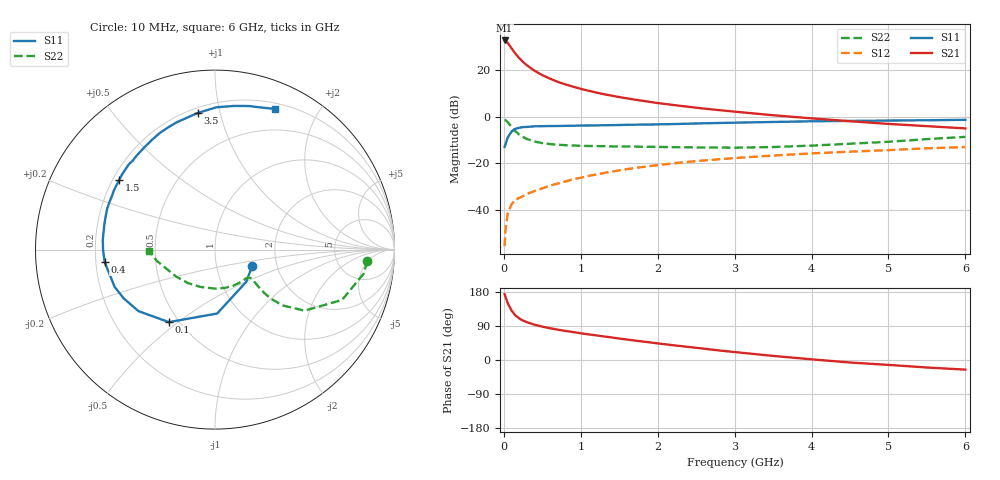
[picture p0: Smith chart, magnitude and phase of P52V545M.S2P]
! SIEMENS Small Signal Semiconductors
! BFP183
! Si NPN RF Bipolar Junction Transistor in SOT143
! VCE = 2.5 V  IC = 45 mA
! Common Emitter S-Parameters:  March  1996
# GHz  S  MA  R  50
!  f  S11  S21  S12  S22
! GHz  MAG  ANG  MAG  ANG  MAG  ANG  MAG  ANG
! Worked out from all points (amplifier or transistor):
!   36 points, 10 MHz to 6 GHz, reference 50 ohm
!   highest |S21| = 32.5 dB at 10 MHz (marker M1)
!   |S21| within 3 dB of that: start of sweep to 92.57 MHz
!   unconditionally stable (mu >= 1): start of sweep to 18.27 MHz; 325 MHz to end of sweep
!   at 250 MHz: K = 0.88, MSG = 28.7 dB, |S12| = -34.0 dB
!   at 1.4 GHz: K = 1.40, MAG = 12.5 dB, |S12| = -23.5 dB
!   at 6 GHz: K = 1.09, MAG = 2.2 dB, |S12| = -13.0 dB
!   S11 on the Smith chart (normalised r, x): 10 MHz: 1.49, -0.29; 100 MHz: 0.44, -0.46; 400 MHz: 0.24, -0.05; 1.5 GHz: 0.23, +0.31; 3.5 GHz: 0.23, +0.85; 6 GHz: 0.26, +1.48
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0.01  0.2264 -24.0  42.32 173.6  0.0017 76.9  0.8506 -4.3
0.02  0.2502 -45.8  41.79 167.6  0.0036 69.7  0.8397 -9.1
0.05  0.3565 -88.1  37.76 150.3  0.0085 68.6  0.7616 -21.6
0.1  0.4789 -122.5  28.78 130.3  0.0133 53.8  0.6038 -34.3
0.15  0.5472 -141.2  22.26 117.9  0.0168 50.5  0.4877 -39.6
0.2  0.5771 -152.0  17.81 109.7  0.0182 50.2  0.413 -41.3
0.25  0.5968 -159.7  14.7 103.9  0.02 50.4  0.3659 -41.4
0.3  0.6009 -165.4  12.45 99.8  0.0222 51.4  0.3318 -40.8
0.4  0.619 -173.6  9.535 93.0  0.0256 54.1  0.2926 -39.6
0.5  0.6238 179.9  7.675 88.1  0.0292 55.4  0.2713 -38.9
0.6  0.6276 174.9  6.473 83.8  0.0334 58.1  0.2585 -38.6
0.7  0.6292 170.1  5.524 80.1  0.037 59.5  0.2502 -38.9
0.9  0.6369 162.9  4.35 73.8  0.0458 60.6  0.2408 -40.7
1.1  0.6451 155.7  3.565 67.6  0.054 60.6  0.235 -43.6
1.5  0.6594 144.2  2.61 56.6  0.0708 58.9  0.2298 -51.2
1.8  0.6757 135.1  2.178 48.8  0.0836 56.9  0.226 -58.5
2.2  0.6914 125.1  1.768 39.0  0.0998 53.2  0.2216 -69.0
2.8  0.7292 111.0  1.373 25.1  0.1225 47.3  0.2178 -87.6
3.5  0.767 97.3  1.068 10.8  0.1469 40.6  0.2234 -111.5
4.5  0.8078 82.3  0.796 -6.6  0.1776 30.7  0.2627 -144.7
5.5  0.8343 71.4  0.624 -19.8  0.2098 21.8  0.3297 -168.9
6  0.8519 66.9  0.559 -25.4  0.2229 16.9  0.368 -178.9
